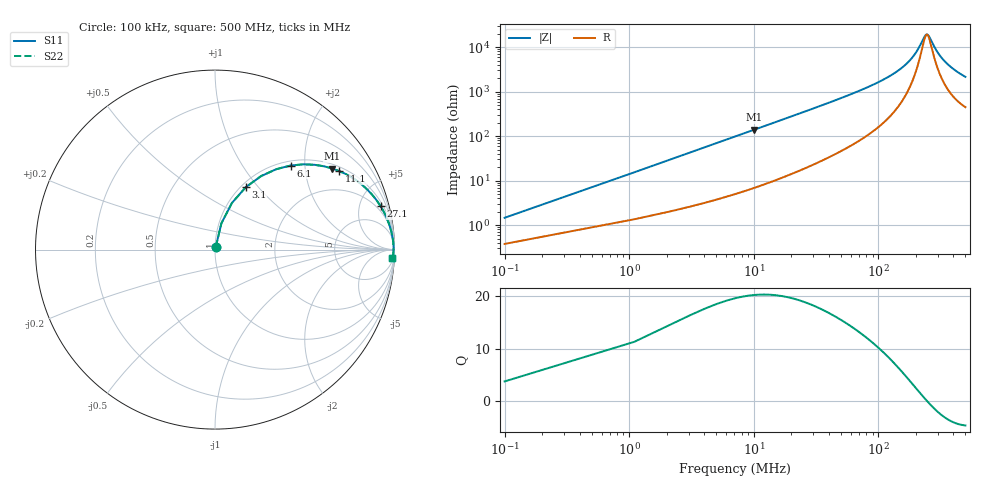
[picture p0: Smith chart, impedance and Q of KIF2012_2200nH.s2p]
!version-2
!date-12.2020
!Series
# MHz S RI R 50
!Freq ReS11 ImS11 ReS21 ImS21 ReS12 ImS12 ReS22 ImS22
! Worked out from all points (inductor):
!   501 points, 100 kHz to 500 MHz, reference 50 ohm
!   read as one part in series: L = 2.21 uH near 2.1 MHz
!   highest Q = 20.2 at 10.1 MHz (marker M1), where L = 2.2 uH
!   self-resonance near 245.8 MHz
!   S11 on the Smith chart (normalised r, x): 100 kHz: 1.01, +0.03; 3.1 MHz: 1.05, +0.86; 6.1 MHz: 1.09, +1.69; 11.1 MHz: 1.15, +3.07; 27.1 MHz: 1.40, +7.52; 500 MHz: 10, -42
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0.1  0.00398 0.014  0.996 -0.014  0.996 -0.014  0.00398 0.014
1.1  0.0356 0.1462  0.9644 -0.1462  0.9644 -0.1462  0.0356 0.1462
3.1  0.1713 0.3476  0.8287 -0.3476  0.8287 -0.3476  0.1713 0.3476
4.1  0.2566 0.4094  0.7434 -0.4094  0.7434 -0.4094  0.2566 0.4094
6.1  0.4207 0.4683  0.5793 -0.4683  0.5793 -0.4683  0.4207 0.4683
10.1  0.6539 0.4517  0.3461 -0.4517  0.3461 -0.4517  0.6539 0.4517
11.1  0.6932 0.4372  0.3068 -0.4372  0.3068 -0.4372  0.6932 0.4372
17.1  0.8362 0.346  0.1638 -0.346  0.1638 -0.346  0.8362 0.346
27.1  0.9228 0.2414  0.0772 -0.2414  0.0772 -0.2414  0.9228 0.2414
37.1  0.9545 0.1813  0.0455 -0.1813  0.0455 -0.1813  0.9545 0.1813
50.1  0.9724 0.1346  0.0276 -0.1346  0.0276 -0.1346  0.9724 0.1346
84.1  0.9877 0.0754  0.0123 -0.0754  0.0123 -0.0754  0.9877 0.0754
167.1  0.9944 0.0233  0.00557 -0.0233  0.00557 -0.0233  0.9944 0.0233
199.1  0.9949 0.0125  0.00513 -0.0125  0.00513 -0.0125  0.9949 0.0125
236.1  0.9949 0.00238  0.00512 -0.00238  0.00512 -0.00238  0.9949 0.00238
243.1  0.9948 0.00065  0.00516 -0.00065  0.00516 -0.00065  0.9948 0.00065
250.1  0.9948 -0.00103  0.00521 0.00103  0.00521 0.00103  0.9948 -0.00103
294.1  0.9943 -0.0106  0.00574 0.0106  0.00574 0.0106  0.9943 -0.0106
334.1  0.9935 -0.0183  0.0065 0.0183  0.0065 0.0183  0.9935 -0.0183
371.1  0.9926 -0.0248  0.00739 0.0248  0.00739 0.0248  0.9926 -0.0248
417.1  0.9913 -0.0323  0.00872 0.0323  0.00872 0.0323  0.9913 -0.0323
500  0.9884 -0.0446  0.0116 0.0446  0.0116 0.0446  0.9884 -0.0446
